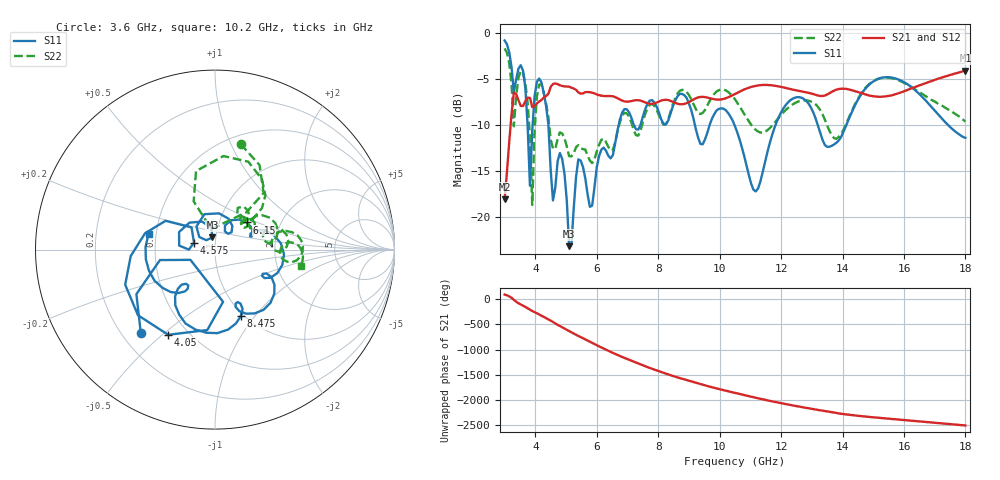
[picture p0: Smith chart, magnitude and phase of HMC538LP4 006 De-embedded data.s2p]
! Chelmsford, MA 01824
! http://www.hittite.com
! Tel: 978-250-3343
! Fax: 978-250-3373
! Device  :  HMC538LP4
! Description:  600 Analog Phase Shifter
! Frequency  :  6.0 GHz - 15.0 GHz
! Package  :  LP4  - 4x4 mm Quad Flatpack No-Lead (QFN) Plastic Package: 24 pin
! Ports  :  2 RF, 1 DC
!  Pin  3  = Rfin  = Port 1
!  Pin  16  = Rfout = Port 2
!  pin  21  = vCTL
! Voltages:  VCTL  = 0 to 5.0 Volts
! Currents :  Vb(V)  Vd(V)  Ib(mA)  Id(mA)
!  0.00  0.60  0.000000	0.484538
! Data:  The device was measured on evaluation board 111296-1.
!  Data was collected using a calibrated network analyzer.
!  The evaluation circuit board was modeled and simulated.This was use
!  to removed the evaluation board circuit from the measured data.
!  The reference plane is the center of the package pin.
! Misc:  Lot #
!Date Measured:  03 - 11 -2009
! Date:  03 - 17 -2009
! Note:
!  Hittite Microwave supplies this data as a sample of measured data at the
!  package pin for this package product.  Your particular data for this product
!  may vary.
!  Data was taken at 25 degrees C.
!  Hittite Microwave reserves the right to change this data at anytime.
# MHz S MA R 50
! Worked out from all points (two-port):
!   201 points, 3 GHz to 18 GHz, reference 50 ohm
!   highest |S21| = -4.12 dB at 18 GHz (marker M1); lowest = -18.0 dB at 3 GHz (marker M2)
!   |S21| within 3 dB of the highest: 4.251 GHz to 6.687 GHz (2.436 GHz wide, 44.5 % of centre); 10.18 GHz to end of sweep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
!   lowest |S11| = -23.1 dB at 5.1 GHz (marker M3), VSWR 1.15, Z = 48.1 + j6.61 ohm
!   |S11| at or under -10 dB: 4.426 GHz to 6.714 GHz (2.288 GHz wide, 41.1 % of centre); 10.48 GHz to 11.82 GHz (1.338 GHz wide, 12 % of centre); 13.19 GHz to 14.12 GHz (932 MHz wide, 6.82 % of centre)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
!   |S22| runs from -18.7 to -1.7 dB; largest |S21 - S12| = 0.0016
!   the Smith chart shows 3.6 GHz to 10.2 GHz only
!   S11 on the Smith chart (normalised r, x): 3.6 GHz: 0.28, -0.42; 4.05 GHz: 0.39, -0.52; 4.575 GHz: 0.79, +0.06; 6.15 GHz: 1.35, +0.43; 8.475 GHz: 0.97, -0.85; 10.2 GHz: 0.45, +0.09
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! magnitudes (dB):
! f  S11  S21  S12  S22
! 3 GHz  -0.9  -18.0  -18.0  -1.7
! 3.3 GHz  -6.4  -6.5  -6.5  -10.1
! 3.6 GHz  -4.1  -7.9  -7.9  -4.4
! 3.825 GHz  -16.6  -7.1  -7.1  -11.3
! 3.9 GHz  -10.6  -8.1  -8.1  -18.7
! 4.05 GHz  -5.3  -7.7  -7.7  -6.9
! 4.575 GHz  -18.2  -5.6  -5.6  -12.6
! 4.875 GHz  -13.7  -5.8  -5.8  -10.9
! 5.1 GHz  -23.1  -5.9  -5.9  -13.4
! 5.55 GHz  -14.5  -6.6  -6.6  -12.6
! 5.85 GHz  -18.7  -6.5  -6.5  -14.1
! 6.15 GHz  -12.7  -6.8  -6.8  -11.6
! 8.025 GHz  -8.7  -7.5  -7.5  -9.0
! 8.475 GHz  -8.0  -7.5  -7.5  -7.8
! 10.2 GHz  -8.4  -7.1  -7.1  -6.3
! 10.5 GHz  -10.1  -6.6  -6.7  -7.2
! 11.18 GHz  -17.2  -5.8  -5.8  -10.5
! 12.15 GHz  -7.9  -6.0  -6.0  -8.4
! 13.05 GHz  -8.7  -6.7  -6.7  -7.6
! 13.8 GHz  -11.9  -6.2  -6.2  -11.5
! 15.53 GHz  -4.8  -6.8  -6.9  -4.9
! 18 GHz  -11.4  -4.1  -4.1  -9.6
